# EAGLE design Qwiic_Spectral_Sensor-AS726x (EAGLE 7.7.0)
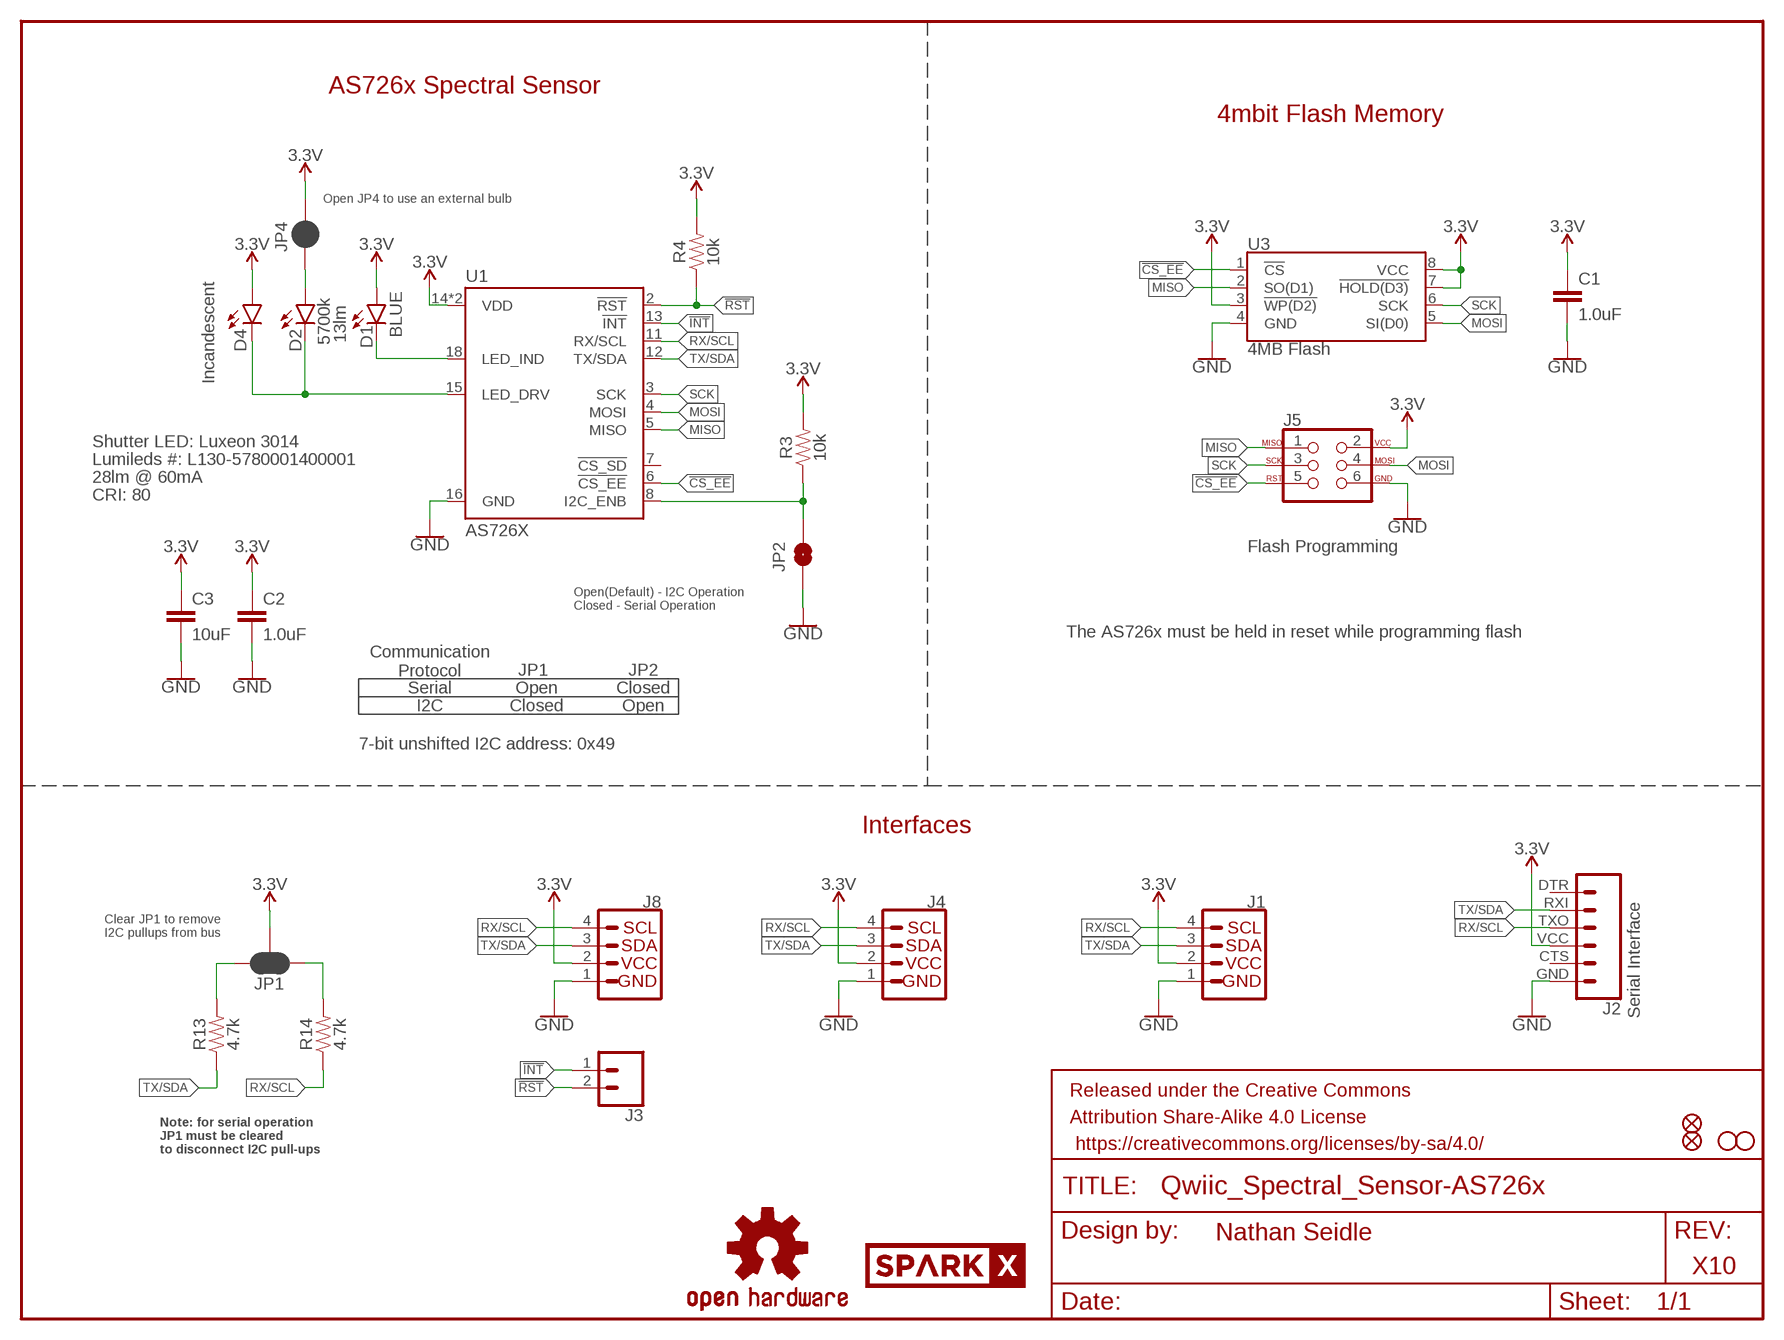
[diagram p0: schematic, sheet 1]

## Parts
C1  1.0uF  1.0UF-0603-16V-10%  [0603]
C2  1.0uF  1.0UF-0603-16V-10%  [0603]
C3  10uF  10UF-0603-6.3V-20%  [0603]
D1  BLUE  LED-BLUE0603  [LED-0603]
D2  5700k  LEDLD  [SUPER_BRIGHT_SMD_LED_1206]
D4  Incandescent  LEDNS  [LED_5MM_NOSILK]
FD1  FIDUCIAL1X2  [FIDUCIAL-1X2]
FD2  FIDUCIAL1X2  [FIDUCIAL-1X2]
FRAME1  FRAME-LETTER  [CREATIVE_COMMONS]
H2  STAND-OFF  [STAND-OFF]
H4  STAND-OFF  [STAND-OFF]
J1  I2C_STANDARDJS-1MM  [1X04_1MM_RA]
J2  Serial Interface  6_PIN_SERIAL_CABLEPTH  [FTDI_BASIC]
J3  CONN_021X02_NO_SILK  [1X02_NO_SILK]
J4  I2C_STANDARDJS-1MM  [1X04_1MM_RA]
J5  Flash Programming  AVR_SPI_PROG_3X2TESTPOINTS  [2X3_TEST_POINTS]
J8  I2C_STANDARD_NO_SILK  [1X04_NO_SILK]
JP1  JUMPER-SMT_3_2-NC_PASTE_SILK  [SMT-JUMPER_3_2-NC_PASTE_SILK]
JP2  JUMPER-SMT_2_NO_SILK  [SMT-JUMPER_2_NO_SILK]
JP4  JUMPER-SMT_2_NC_PASTE_NO-SILK  [SMT-JUMPER_2_NC_PASTE_NO-SILK]
LOGO4  OSHW-LOGOS  [OSHW-LOGO-S]
R3  10k  10KOHM-0603-1/10W-1%  [0603]
R4  10k  10KOHM-0603-1/10W-1%  [0603]
R13  4.7k  4.7KOHM-0603-1/10W-1%  [0603]
R14  4.7k  4.7KOHM-0603-1/10W-1%  [0603]
U1  AS726X  [LGA20]
U3  4MB Flash  AT25SF041  [SO08]
U$1  SPARKX-LOGO3  [SPARKX-SMALL]

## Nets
3.3V: C1.1 C2.1 C3.1 D1.A D4.A J1.2(VCC) J2.VCC J4.2(VCC) J5.2 J8.2 JP1.2 JP4.2 R3.2 R4.2 U1.14(VDD) U1.17(VDD) U3.3(!WP(D2)) U3.7(!HOLD(D3)) U3.8(VCC)
!CS_EE: J5.5 U1.6(!CS_EE) U3.1(!CS)
!INT: J3.1 U1.13(!INT)
!RST: J3.2 R4.1 U1.2(!RST)
GND: C1.2 C2.2 C3.2 J1.1(GND) J2.GND J4.1(GND) J5.6 J8.1 JP2.1 U1.16(GND) U3.4(GND)
LED_DRV: D2.C D4.K(C) U1.15(LED_DRV)
MISO: J5.1 U1.5(MISO) U3.2(SO(D1))
MOSI: J5.4 U1.4(MOSI) U3.5(SI(D0))
N$1: JP2.2 R3.1 U1.8(I2C_ENB)
N$2: D1.C U1.18(LED_IND)
N$4: JP1.3 R13.2
N$5: JP1.1 R14.2
N$6: D2.A JP4.1
RX/SCL: J1.4(SCL) J2.TXO J4.4(SCL) J8.4 R14.1 U1.11(RX/SCL)
SCK: J5.3 U1.3(SCK) U3.6(SCK)
TX/SDA: J1.3(SDA) J2.RXI J4.3(SDA) J8.3 R13.1 U1.12(TX/SDA)
Unconnected: J2.CTS J2.DTR U1.7(!CS_SD)

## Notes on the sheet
- AS726x Spectral Sensor
- 4mbit Flash Memory
- Open JP4 to use an external bulb
- 13lm
- Shutter LED: Luxeon 3014
- Lumileds #: L130-5780001400001
- 28lm @ 60mA
- CRI: 80
- Open(Default) - I2C Operation
  Closed - Serial Operation
- The AS726x must be held in reset while programming flash
- Communication
  Protocol
- JP1 | JP2
- Serial | Open | Closed
- I2C | Closed | Open
- 7-bit unshifted I2C address: 0x49
- Interfaces
- Clear JP1 to remove
  I2C pullups from bus
- Note: for serial operation
  JP1 must be cleared
  to disconnect I2C pull-ups
- Nathan Seidle
- X10

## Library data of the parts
C1 C2 = SparkFun-Capacitors:1.0UF: 1µF ceramic capacitors; PROD_ID: CAP-00868
C3 = SparkFun-Capacitors:10UF: 10.0µF ceramic capacitors; PROD_ID: CAP-11015
D1 = SparkFun-LED:LED-BLUE: Blue SMD LED; PROD_ID: DIO-08575
D2 D4 = SparkX:LED
FD1 FD2 = SparkFun-Aesthetics:FIDUCIAL: Fiducial Alignment Points
FRAME1 = SparkFun-Aesthetics:FRAME-LETTER: Schematic Frame - Letter
H2 H4 = SparkFun-Hardware:STAND-OFF: Stand Off
J1 J4 = SparkX:I2C_STANDARD: SparkFun I2C Standard Pinout Header SparkFun has standardized on a pinout for all I2C based sensor breakouts. This pinout allows I2C boards to be plugged directly into the headers on Arduino Uno compatible boards, and to be daisy chained easily. Example SparkFun Products: SparkFun Atmospheric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
J2 = SparkFun-Connectors:6_PIN_SERIAL_CABLE: 6-pin header connection for use with the "FTDI BASIC" pinout - CABLE SIDE. Also known as "Arduino Serial Program Header". This is used on a design to provide a 6-pin connection point for serial communication usually from a USB cable (D+/D-) to these headers (RX/TX). It also has the remaining pins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
J3 = SparkFun-Connectors:CONN_02: Multi connection point. Often used as Generic Header-pin footprint for 0.1 inch spaced/style header connections
J5 = SparkFun-Connectors:AVR_SPI_PROG_3X2: AVR ISP 6 Pin This is the reduced ISP connector for AVR programming. Common on Arduino. This footprint will take up less PCB space and can be used with a 10-pin to 6-pin adapter such as SKU: BOB-08508 **Special note about "TEST_POINT" package. The stop mask is on the top side, so if you want your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
J8 = SparkFun-Connectors:I2C_STANDARD: SparkFun I2C Standard Pinout Header SparkFun has standardized on a pinout for all I2C based sensor breakouts. This pinout allows I2C boards to be plugged directly into the headers on Arduino Uno compatible boards, and to be daisy chained easily. Example SparkFun Products: SparkFun Atmospheric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
JP1 = SparkFun-Jumpers:JUMPER-SMT_3_2-NC_PASTE: Normally closed solder jumper (2 of 2 connections) This jumper has an aperture in the stencil to allow solder paste to bridge both connections. Both connections are normally closed (NC). Wick off the solder to open the connection(s). Reapply solder to reclose the connection(s).
JP2 = SparkFun-Jumpers:JUMPER-SMT_2_NO: Normally open jumper
JP4 = SparkFun-Jumpers:JUMPER-SMT_2_NC_PASTE: Normally closed solder jumper
LOGO4 = SparkFun-Aesthetics:OSHW-LOGO: Open-Source Hardware (OSHW) Logo
R3 R4 = SparkFun-Resistors:10KOHM: 10kΩ resistor; PROD_ID: RES-00824
R13 R14 = SparkFun-Resistors:4.7KOHM: 4.7kΩ resistor; PROD_ID: RES-07857
U1 = SparkX:AS726X
U3 = SparkFun-IC-Memory:AT25SF041: AT25SF041 4Mb Serial Flash Memory 104MHz, SPI, 8-SOIC Datasheet SparkFun Products: SparkFun ESP8266 Thing SparkFun ESP8266 Thing - Dev Board; PROD_ID: IC-12455
U$1 = SparkX:SPARKX-LOGO

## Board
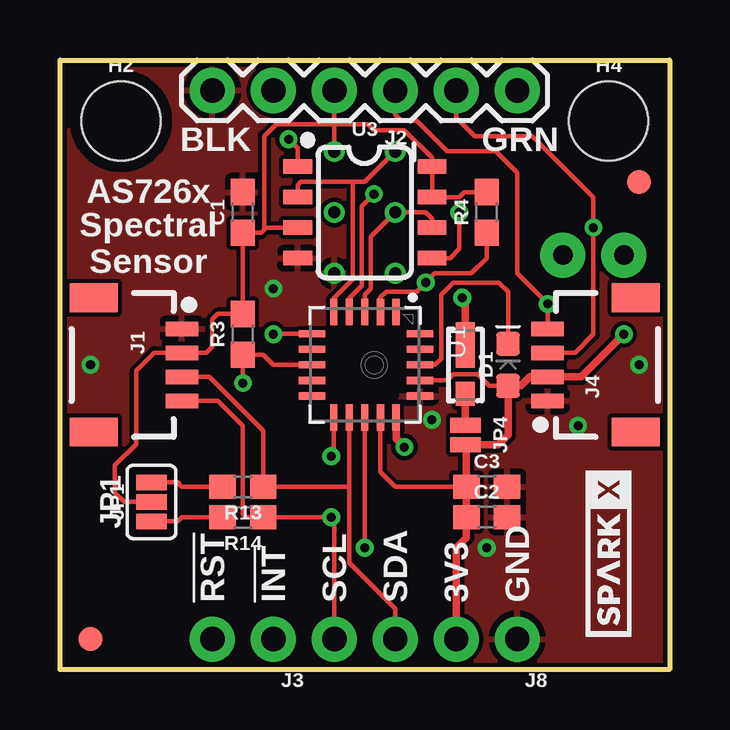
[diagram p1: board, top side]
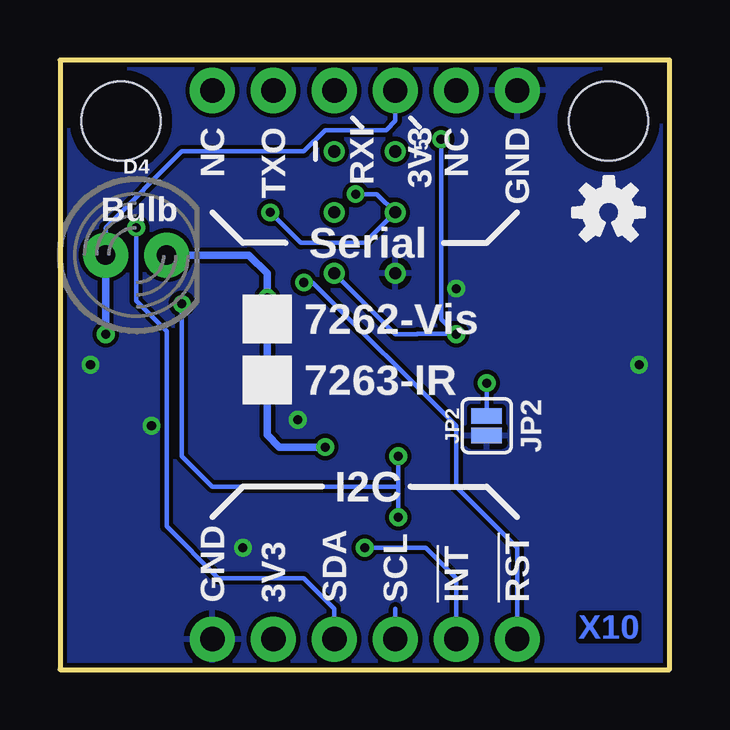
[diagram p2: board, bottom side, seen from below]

Size 25.4 x 25.4 mm. Coordinates in mm from the lower left corner, seen from the top.
Outline: 0,0 0,25.4 25.4,25.4 25.4,0 0,0
Copper layers (1*16): Top 0.035mm / dielectric 1.5mm / Bottom 0.035mm
Design rules "SparkFun-2-layer-TIGHT": minimum track width 7mil, minimum drill 15mil, track to track 7mil, track to pad 7mil, pad to pad 7mil, via to via 7mil, smd to smd 7mil, copper to edge 7mil, drill to drill 7mil, minimum pad ring 7mil, minimum via ring 7mil, stop-mask expansion 4mil, vias tented up to drill 25mil, thermal gap 10mil

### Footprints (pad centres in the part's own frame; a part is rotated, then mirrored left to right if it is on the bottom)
0603 = smd 1.1 x 1: 1 -0.85,0; 2 0.85,0
LED-0603 = smd 1 x 1: A -0.877,0; C 0.877,0
SUPER_BRIGHT_SMD_LED_1206 = smd 1 x 0.8: A -1.2,0 | smd 1.9 x 0.8: C 0.827,0
LED_5MM_NOSILK = drill 0.813 pad 1.88: A -1.27,0; K 1.27,0
FIDUCIAL-1X2 = smd 1 x 1: 1 0,0
STAND-OFF = hole 3.302: 0,0
1X04_1MM_RA = smd 0.6 x 1.35: 1 -1.5,0; 2 -0.5,0; 3 0.5,0; 4 1.5,0 | smd 1.2 x 2: NC1 2.8,-3.675; NC2 -2.8,-3.675
FTDI_BASIC = drill 1.016 pad 1.88: CTS 10.16,0; DTR 0,0; GND 12.7,0; RXI 2.54,0; TXO 5.08,0; VCC 7.62,0
1X02_NO_SILK = drill 1.016 pad 1.88: 1 0,0; 2 2.54,0
2X3_TEST_POINTS = drill 0.508: 1 -2.54,-1.27; 2 -2.54,1.27; 3 0,-1.27; 4 0,1.27; 5 2.54,-1.27; 6 2.54,1.27
1X04_NO_SILK = drill 1.016 pad 1.88: 1 0,0; 2 2.54,0; 3 5.08,0; 4 7.62,0
SMT-JUMPER_3_2-NC_PASTE_SILK = smd 0.635 x 1.27: 1 -0.813,0; 2 0,0; 3 0.813,0
SMT-JUMPER_2_NO_SILK = smd 0.635 x 1.27: 1 -0.406,0; 2 0.406,0
SMT-JUMPER_2_NC_PASTE_NO-SILK = smd 0.635 x 1.27: 1 -0.406,0; 2 0.406,0
LGA20 = smd 1.1 x 0.3: 1 -2.2,1.3; 2 -2.2,0.65; 3 -2.2,0; 4 -2.2,-0.65; 5 -2.2,-1.3; 11 2.2,-1.3; 12 2.2,-0.65; 13 2.2,0; 14 2.2,0.65; 15 2.2,1.3 | smd 0.3 x 1.1: 6 -1.3,-2.2; 7 -0.65,-2.2; 8 0,-2.2; 9 0.65,-2.2; 10 1.3,-2.2; 16 1.3,2.3; 17 0.65,2.3; 18 0,2.3; 19 -0.65,2.3; 20 -1.3,2.3
SO08 = smd 0.6 x 1.2: 1 -1.905,-2.8; 2 -0.635,-2.8; 3 0.635,-2.8; 4 1.905,-2.8; 5 1.905,2.8; 6 0.635,2.8; 7 -0.635,2.8; 8 -1.905,2.8

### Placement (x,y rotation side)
C1  7.62,19.05 90 top
C2  17.78,6.35 0 top
C3  17.78,7.62 0 top
D1  18.67,12.7 90 top
D2  16.89,12.7 90 top
D4  22.23,17.27 0 bottom
FD1  1.27,1.27 0 top
FD2  24.13,20.32 0 top
FRAME1  not placed on the board
H2  2.54,22.86 0 top
H4  22.86,22.86 0 top
J1  5.08,12.7 270 top
J2  19.05,24.13 180 top
J3  8.89,1.27 180 top
J4  20.32,12.7 90 top
J5  12.7,19.05 270 bottom
J8  19.05,1.27 180 top
JP1  3.81,6.99 90 top
JP2  7.62,10.16 90 bottom
JP4  16.89,9.78 270 top
LOGO4  2.54,19.05 0 bottom
R3  7.62,13.97 90 top
R4  17.78,19.05 90 top
R13  7.62,7.62 180 top
R14  7.62,6.35 180 top
U1  12.7,12.7 270 top
U3  12.7,19.05 270 top
U$1  22.86,4.83 90 top

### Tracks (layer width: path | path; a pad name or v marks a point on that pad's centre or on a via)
3.3V  (via drill 0.38)
  Top 0.178: C3.1 13.97,7.62 13.35,8.24 U1.14 | U3.3 8.6,18.41 8.51,18.33 | R4.2 16.85,19.9 16.64,19.68 U3.7 U3.8 15.5,21.33 14.35,22.48 13.08,22.48 12.83,22.73 11.43,22.73 | 8.51,18.33 8.51,22.23 9.02,22.73 11.43,22.73 | 8.51,18.33 8.38,18.2 C1.1 R3.2 6.57,14.82 6.35,14.61 6.35,13.46 6.09,13.2 J1.2 3.94,13.21 3.17,12.45 3.17,9.4 2.29,8.51 2.29,7.37 2.67,6.99 JP1.2 | J2.VCC 11.43,22.73 | 11.43,22.73 J5.2 | J4.2 | U1.17 16.13,12.05 16.38,12.31 17.4,12.31 17.88,11.82 D1.A
  Top 0.305: J8.2 16.51,5.08 16.93,5.5 C2.1 C3.1 16.93,9.33 JP4.2 18.26,9.37 18.67,9.78 D1.A 19.19,11.82 19.57,12.2 J4.2 21.73,12.2 v23.5,13.97
  Bottom 0.178: D4.A 23.5,18.41 20.32,21.59 15.24,21.59 14.35,22.48 11.81,22.48 11.43,22.86 J2.VCC
  Bottom 0.305: v23.5,13.97 D4.A
!CS_EE  (via drill 0.38)
  Top 0.178: U3.1 9.9,21.72 v9.53,22.1 | U1.6 8.92,14 v8.89,13.97
  Bottom 0.178: v9.53,22.1 9.53,14.61 v8.89,13.97 8.92,14 U1.6 10.53,13.97 11.43,13.97 J5.5
!INT  (via drill 0.38)
  Top 0.178: U1.13 v12.7,5.08
  Bottom 0.178: J3.1 8.89,3.81 10.16,5.08 v12.7,5.08
!RST  (via drill 0.38)
  Top 0.178: U1.2 13.35,15.51 13.59,15.75 14.86,15.75 v15.24,16.13 15.62,16.51 17.14,16.51 17.78,17.14 R4.1
  Bottom 0.178: v15.24,16.13 14.86,16.13 8.89,10.16 8.89,7.62 6.35,5.08 J3.2
GND  (via drill 0.38)
  other vias: 15.49,10.41 8.89,15.88 1.27,12.7 24.13,12.7 21.59,10.16 17.78,5.08
  pour Top (isolate 0.178): 0,0 25.4,0 25.4,25.4 0,25.4
  pour Bottom (isolate 0.178): 0,25.4 25.4,25.4 25.4,0 0,0
LED_DRV  (via drill 0.38)
  Top 0.305: U1.15 14,9.62 v14.35,9.27 | D2.C 16.89,15.37 v16.76,15.49
  Bottom 0.305: v14.35,9.27 16.26,9.27 16.76,9.78 v16.76,15.49 16.76,16.51 17.53,17.27 D4.K
MISO
  Top 0.178: 12.19,20.32 12.19,16.26 11.4,15.46 U1.5 | U3.2 9.9,20.19 10.03,20.32 12.19,20.32 | 12.19,20.32 12.7,20.32 J5.1
MOSI  (via drill 0.38)
  Top 0.178: U1.4 12.05,15.48 12.57,16 12.57,19.3 v13.08,19.81 | U3.5 16.26,17.14 16.64,17.53 v16.64,19.05
  Bottom 0.178: v13.08,19.81 12.19,19.81 J5.4 12.7,17.78 15.37,17.78 v16.64,19.05
N$1  (via drill 0.38)
  Top 0.178: U1.8 8.89,12.7 8.47,13.12 R3.1 v7.62,11.94
  Bottom 0.178: v7.62,11.94 JP2.2
N$2
  Top 0.178: U1.18 15.62,12.7 15.88,12.95 15.88,15.62 16.38,16.13 18.29,16.13 18.67,15.75 D1.C
N$4
  Top 0.178: R13.2 5.08,7.62 4.9,7.8 JP1.3
N$5
  Top 0.178: R14.2 5.08,6.35 4.9,6.17 JP1.1
N$6
  Top 0.305: JP4.1 D2.A
RX/SCL  (via drill 0.38)
  Top 0.178: J4.4 v20.32,15.24 19.05,16.51 19.05,20.7 18.16,21.59 16.13,21.59 14.86,22.86 14.22,22.86 13.97,23.11 J2.TXO | J1.4 6.58,11.2 7.62,10.16 7.62,6.48 7.75,6.35 R14.1 v11.3,6.35 11.43,6.22 J8.4 | U1.11 11.4,8.99 v11.3,8.89
  Bottom 0.178: 11.3,7.62 19.05,7.62 20.32,8.89 v20.32,15.24 | J8.4 11.43,2.54 | v11.3,6.35 11.3,7.62 | 11.3,7.62 v11.3,8.89
SCK
  Top 0.178: U1.3 12.7,15.62 12.95,15.88 12.95,18.03 J5.3 15.24,19.05 15.5,18.79 U3.6
TX/SDA  (via drill 0.38)
  Top 0.178: U1.12 12.05,7.62 | 12.05,7.62 12.05,4.46 13.97,2.54 J8.3 | J2.RXI 16.51,22.99 17.27,22.23 19.68,22.23 22.23,19.68 v22.23,18.41 22.23,13.97 21.46,13.21 J4.3 | 12.05,7.62 R13.1 8.47,9.95 6.21,12.2 J1.3
  Bottom 0.178: J8.3 13.97,2.54 15.24,3.81 18.8,3.81 20.95,5.97 20.95,14.1 22.23,15.37 v22.23,18.41

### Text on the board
Bottom: X10
tPlace: BLK | GRN | AS726x | Spectral / Sensor | JP1 | !RST | !INT | SCL | SDA | 3V3 | GND
bPlace: GND | NC | 3V3 | RXI | TXO | NC | Bulb | Serial | 7262-Vis | 7263-IR | JP2 | I2C | !RST | !INT | SCL | SDA | 3V3 | GND
tValues: 5700K
tDocu: Nathan Seidle

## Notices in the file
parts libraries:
SparkFun-Aesthetics: Licensing: Creative Commons ShareAlike 4.0 International - https://creativecommons.org/licenses/by-sa/4.0
SparkFun-Aesthetics: Released under the Creative Commons Attribution Share-Alike 4.0 License
SparkFun-Aesthetics: https://creativecommons.org/licenses/by-sa/4.0
